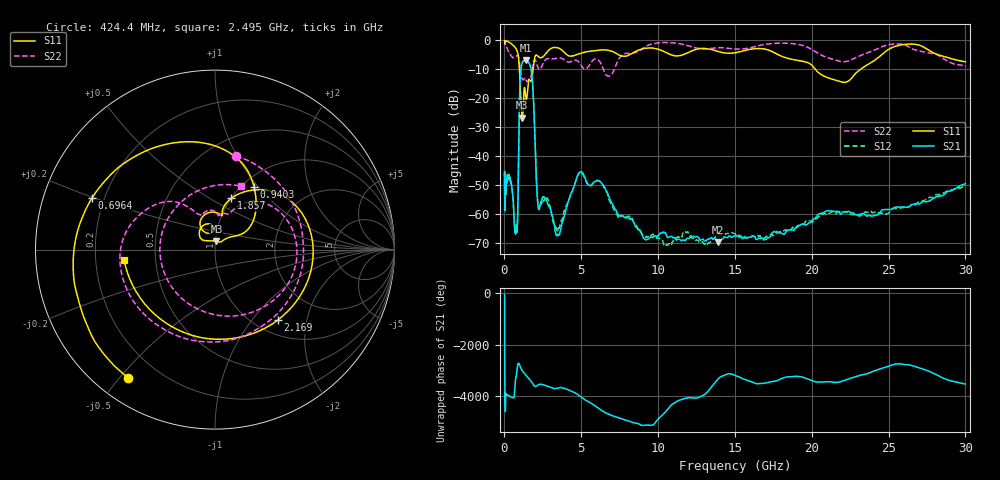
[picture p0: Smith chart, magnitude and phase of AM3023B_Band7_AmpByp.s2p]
# Hz S DB R 50.0
!freq dBS11 angS11 dBS21 angS21 dBS12 angS12 dBS22 angS22
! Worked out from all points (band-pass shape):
!   1601 points, 10 MHz to 30 GHz, reference 50 ohm
!   highest |S21| = -7.09 dB at 1.396 GHz (marker M1); lowest = -69.6 dB at 13.88 GHz (marker M2)
!   |S21| within 3 dB of the highest: 1.069 GHz to 1.734 GHz (665.1 MHz wide, 47.4 % of centre)
!   lowest |S11| = -26.8 dB at 1.143 GHz (marker M3), VSWR 1.10, Z = 50.6 + j4.59 ohm
!   |S11| at or under -10 dB: 971.1 MHz to 1.867 GHz (896.2 MHz wide, 63.1 % of centre); 20.21 GHz to 23.21 GHz (2.998 GHz wide, 13.8 % of centre)
!   |S22| runs from -14.4 to -0.9 dB; largest |S21 - S12| = 0.0083
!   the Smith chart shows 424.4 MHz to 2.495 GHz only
!   S11 on the Smith chart (normalised r, x): 424.4 MHz: 0.09, -0.52; 696.4 MHz: 0.15, +0.20; 940.3 MHz: 1.13, +0.95; 1.857 GHz: 1.00, +0.63; 2.169 GHz: 1.26, -1.36; 2.495 GHz: 0.33, -0.05
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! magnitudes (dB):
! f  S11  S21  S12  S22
! 10 MHz  -0.4  -48.7  -47.0  -0.9
! 38.04 MHz  -0.2  -58.7  -57.2  -1.0
! 144.7 MHz  -0.4  -48.8  -48.2  -2.5
! 424.4 MHz  -1.3  -49.2  -48.9  -5.4
! 547.7 MHz  -1.8  -54.4  -54.4  -6.1
! 696.4 MHz  -2.6  -65.4  -66.7  -5.9
! 838.1 MHz  -4.0  -63.5  -64.2  -5.4
! 940.3 MHz  -7.7  -32.6  -32.2  -6.6
! 1.019 GHz  -15.9  -13.8  -13.8  -10.0
! 1.143 GHz  -26.8  -8.1  -8.0  -13.2
! 1.396 GHz  -20.3  -7.1  -7.1  -13.7
! 1.857 GHz  -10.4  -17.2  -17.1  -8.4
! 2.084 GHz  -5.2  -49.0  -48.7  -7.9
! 2.169 GHz  -5.6  -56.4  -56.2  -9.4
! 2.495 GHz  -5.8  -54.2  -55.7  -8.3
! 3.489 GHz  -2.8  -67.3  -64.9  -6.3
! 4.977 GHz  -4.6  -45.4  -45.6  -8.7
! 7.926 GHz  -5.6  -61.3  -60.9  -4.6
! 13.88 GHz  -4.0  -69.6  -67.5  -2.7
! 21.67 GHz  -14.1  -59.0  -59.5  -7.2
! 25.95 GHz  -1.6  -57.5  -57.8  -1.6
! 30 GHz  -7.5  -49.6  -50.2  -9.1
